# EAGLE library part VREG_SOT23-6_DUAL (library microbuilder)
Dual Output SOT23-6 Linear Regulators Diodes Inc. AP7312 - Dual 150mA LDO Linear Regulator 0.2V dropout, 150mA output, 2-6V Input AP7312-1833W6-7 - 1.8V/3.3V SOT23-6 (Digikey: AP7312-1833W6-7DICT-ND) MIC5320 - Dual 150mA ULDO Linear Regulator Ultra-low 35mV dropout at 150mA, 2.3-5.5V Input 3.3V/1.8V SOT23-6 (Digikey: 576-1658-1-ND) 3.3V/1.5V SOT23-6 (Digikey: 576-3483-1-ND)
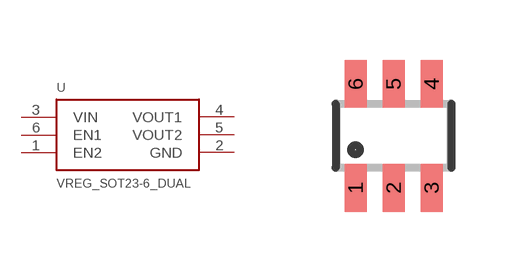
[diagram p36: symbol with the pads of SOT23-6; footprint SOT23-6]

Designator prefix U

## VREG_SOT23-6_DUALMIC5320  [SOT23-6]
1  EN2
2  GND
3  VIN
4  VOUT1
5  VOUT2
6  EN1

## VREG_SOT23-6_DUALAP7312  [SOT23-6]
1  VOUT2
2  GND
3  EN2
4  EN1
5  VIN
6  VOUT1

## Footprint SOT23-6 (pad centres in mm)
Small Outline Transistor - 6 Pin
smd 0.55 x 1.2: 1 -0.95,-1.3; 2 0,-1.3; 3 0.95,-1.3; 4 0.95,1.3; 5 0,1.3; 6 -0.95,1.3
